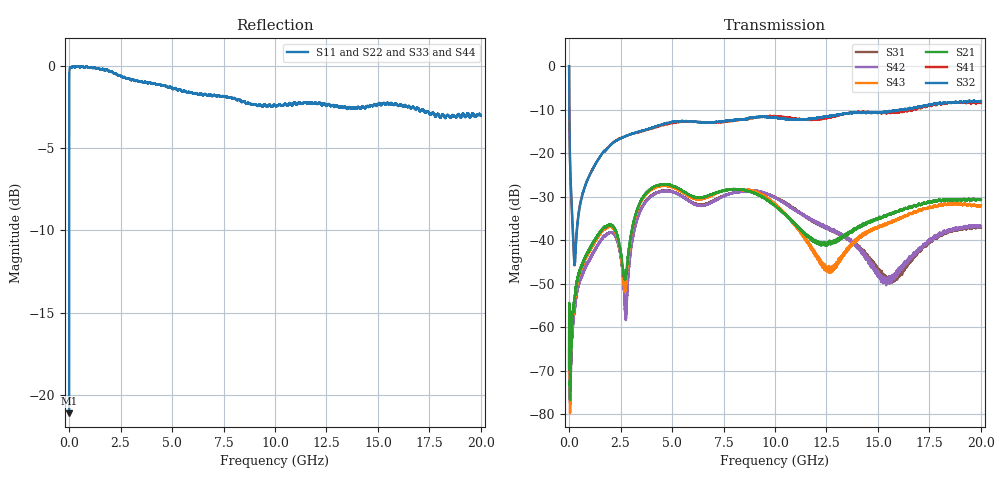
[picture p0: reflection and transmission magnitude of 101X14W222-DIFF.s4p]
!{101X14W222}
!Johanson Technology Inc.
!www.johansontechnology.com
!Test Board Conditions:
!Substrate Type  RO4350B
!Substrate Thickness  10 mil
!Substrate Dk  3.66
!TL Type: GCPW
!TL Trace Width  20 mil
!TL Gap  15 mil
!PART MODE DIFFERENTIAL
!DUT TOPOLOGY	DIFFERENTIAL 4-PORT
!Mounting Pad LxW  20x35 mil
# MHz S  dB  R 50
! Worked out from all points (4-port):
!   20001 points, 300 kHz to 20 GHz, reference 50 ohm
!   strongest paths, dB at 300 kHz, 5 GHz, 10 GHz, 15 GHz, 20 GHz:
!     S32: 0.0, -12.8, -11.9, -10.7, -8.0
!     S41: -0.1, -13.1, -11.5, -10.7, -8.5
!     S21: -69.6, -27.5, -32.1, -35.1, -30.8
!     S43: -67.7, -27.8, -31.6, -36.9, -32.1
!     S42: -70.8, -28.9, -30.2, -47.7, -36.8
!     S31: -69.2, -28.8, -30.2, -46.9, -37.0
!   lowest |S11| = -21.1 dB at 300 kHz (marker M1), VSWR 1.19, Z = 48.5 - j8.56 ohm
!   |S11| at or under -10 dB: start of sweep to 1.229 MHz
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0.3  -21.12 -95.0  -68.64 105.2  -67.24 54.9  -0.04 -5.2
     -69.62 74.1  -21.49 -96.9  -0.02 -4.8  -72.13 67.9
     -69.20 65.1  -0.01 -4.7  -21.41 -96.0  -69.01 85.2
     -0.06 -5.2  -70.77 96.7  -67.74 58.4  -21.11 -94.5
279.296  -0.07 178.2  -52.67 79.9  -55.28 78.2  -45.23 18.8
         -52.51 79.5  -0.07 178.3  -45.34 12.3  -55.20 81.7
         -55.63 78.6  -45.36 12.6  -0.05 178.4  -53.67 79.8
         -45.15 20.4  -55.14 81.0  -53.35 80.2  -0.03 177.9
2010.27  -0.35 162.8  -36.46 38.5  -38.21 27.9  -18.06 59.3
         -36.43 38.3  -0.33 162.4  -18.15 59.5  -38.24 27.9
         -38.21 27.9  -18.16 59.5  -0.29 163.8  -36.81 38.3
         -18.11 59.3  -38.24 28.2  -36.85 38.4  -0.32 164.2
2757.259  -0.73 160.0  -48.01 82.9  -57.80 -138.0  -16.04 45.1
          -47.78 82.5  -0.66 158.7  -16.11 45.8  -57.34 -131.7
          -56.97 -134.7  -16.09 45.9  -0.67 159.7  -49.98 90.3
          -16.05 45.3  -57.70 -131.8  -50.06 89.8  -0.70 161.0
4312.235  -1.13 149.0  -27.38 48.9  -28.98 45.5  -13.89 32.1
          -27.43 49.0  -1.14 151.1  -13.75 32.7  -29.03 47.2
          -28.97 45.2  -13.72 32.7  -1.15 151.8  -27.64 51.5
          -13.93 31.9  -29.04 46.9  -27.70 51.2  -1.07 153.3
12621.11  -2.34 107.8  -40.68 -16.3  -37.36 -108.8  -11.67 -13.5
          -40.50 -16.3  -2.44 110.2  -11.40 -14.6  -37.08 -105.2
          -37.27 -106.4  -11.50 -14.2  -2.17 115.5  -46.84 -19.4
          -11.72 -13.4  -37.43 -104.8  -46.87 -19.1  -2.12 121.8
20000  -3.04 61.9  -30.78 -38.5  -37.01 -71.4  -8.46 -45.8
       -30.77 -38.6  -3.27 61.5  -8.05 -48.0  -36.74 -69.7
       -37.04 -70.6  -8.04 -46.9  -3.04 68.8  -32.02 -26.6
       -8.47 -45.3  -36.81 -69.8  -32.11 -26.6  -2.81 73.2
